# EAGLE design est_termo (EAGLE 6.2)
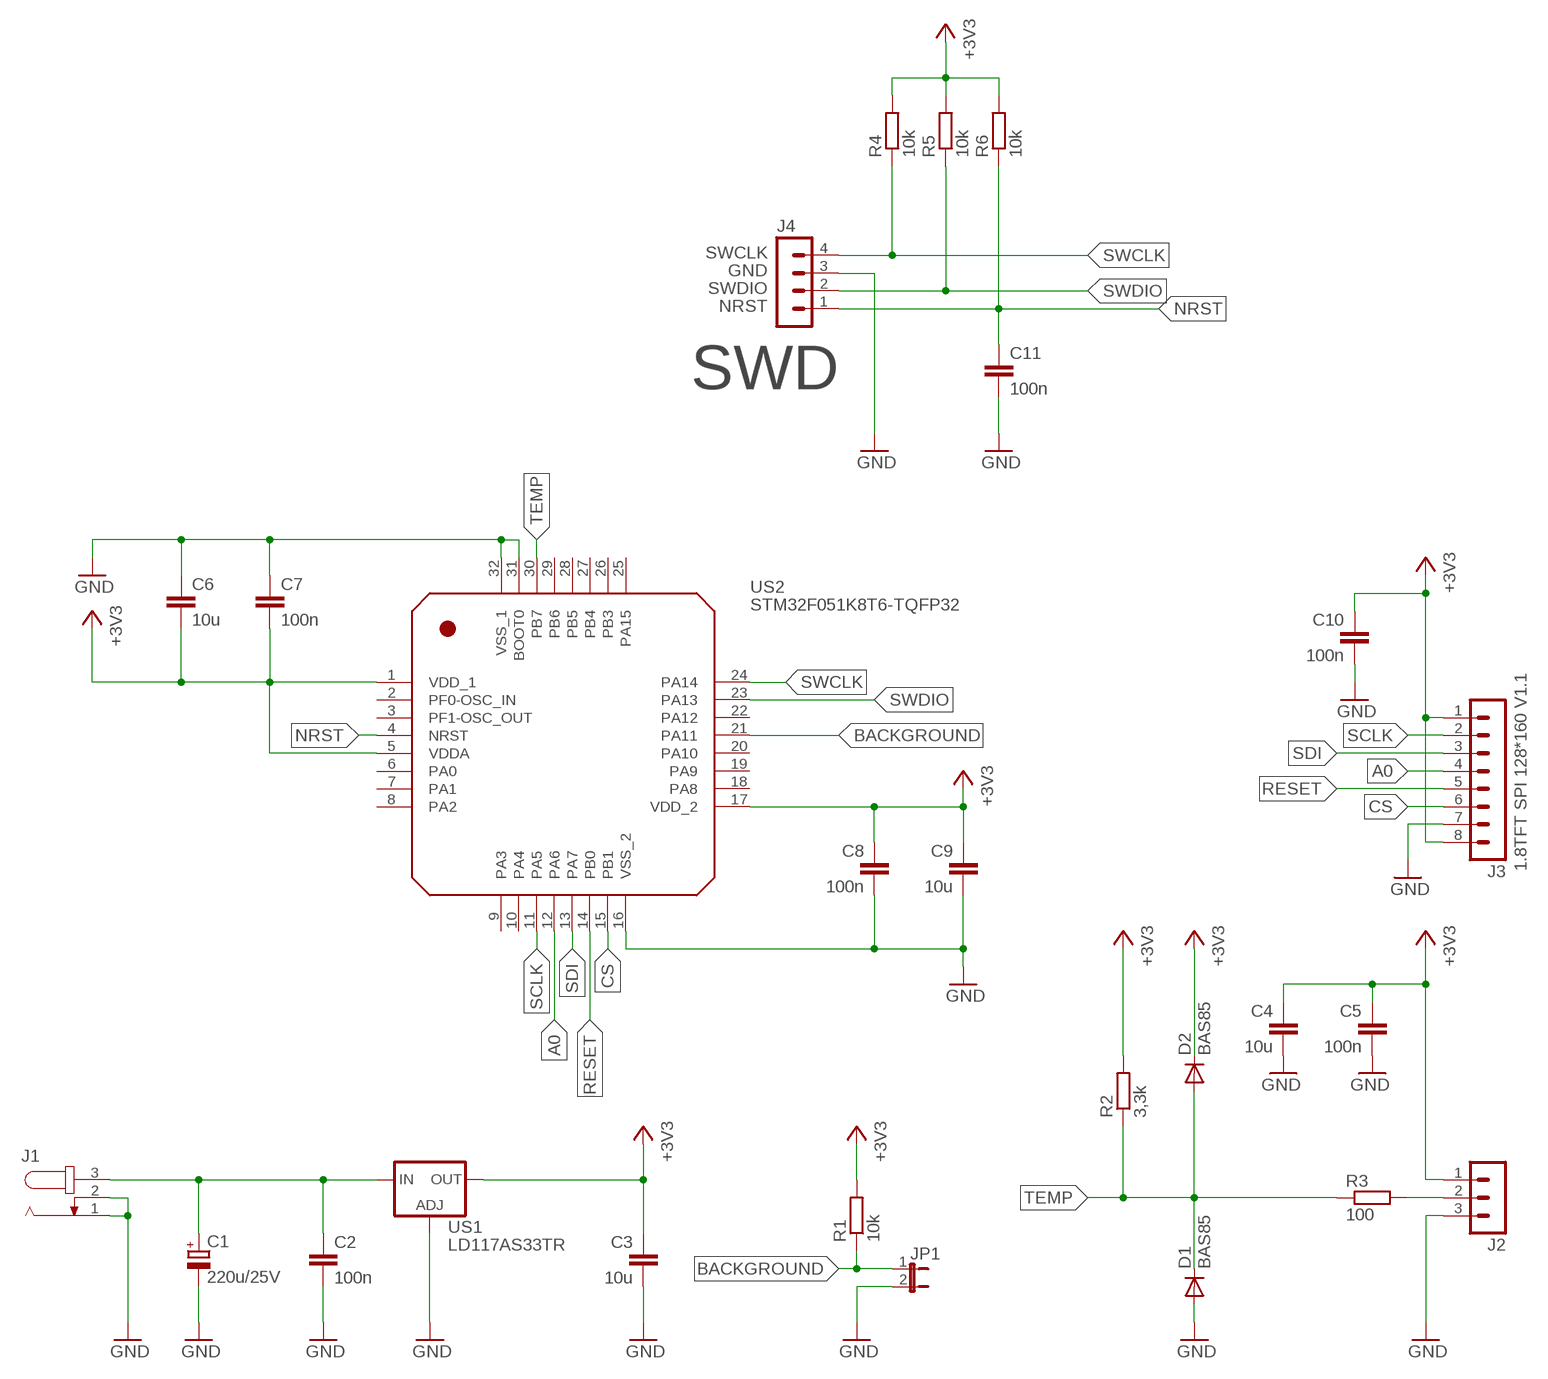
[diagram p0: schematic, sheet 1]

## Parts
C1  220u/25V  CPOL-EUTT2D7L  [TT2D7L]
C2  100n  C-EUC0805  [C0805]
C3  10u  C-EUC0805  [C0805]
C4  10u  C-EUC0805  [C0805]
C5  100n  C-EUC0805  [C0805]
C6  10u  C-EUC0805  [C0805]
C7  100n  C-EUC0805  [C0805]
C8  100n  C-EUC0805  [C0805]
C9  10u  C-EUC0805  [C0805]
C10  100n  C-EUC0805  [C0805]
C11  100n  C-EUC0805  [C0805]
D1  BAS85  DIODE-MINIMELF  [MINIMELF]
D2  BAS85  DIODE-MINIMELF  [MINIMELF]
J1  JACK-PLUG0  [SPC4077]
J2  MA03-1  [MA03-1]
J3  1.8TFT SPI 128*160 V1.1  MA08-1  [MA08-1]
J4  MA04-1  [MA04-1]
JP1  JP1E  [JP1]
R1  10k  R-EU_R0805  [R0805]
R2  3,3k  R-EU_R0805  [R0805]
R3  100  R-EU_R0805  [R0805]
R4  10k  R-EU_R0805  [R0805]
R5  10k  R-EU_R0805  [R0805]
R6  10k  R-EU_R0805  [R0805]
US1  LD117AS33TR  [SOT223]
US2  STM32F051K8T6-TQFP32  STM32F051-TQFP32  [TQFP32]

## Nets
+3V3: C3.1 C4.1 C5.1 C6.2 C7.2 C8.1 C9.1 C10.1 D2.C J2.1 J3.1 J3.8 R1.2 R2.2 R4.2 R5.2 R6.2 US1.4(OUT) US2.1(VDD_1) US2.5(VDDA) US2.17(VDD_2)
A0: J3.4 US2.12(PA6)
BACKGROUND: JP1.1 R1.1 US2.21(PA11)
CS: J3.6 US2.15(PB1)
GND: C1.- C2.2 C3.2 C4.2 C5.2 C6.1 C7.1 C8.2 C9.2 C10.2 C11.2 D1.A J1.1 J1.2 J2.3 J3.7 J4.3 JP1.2 US1.1(ADJ) US2.16(VSS_2) US2.31(BOOT0) US2.32(VSS_1)
N$1: C1.+ C2.1 J1.3 US1.3(IN)
N$28: J2.2 R3.2
NRST: C11.1 J4.1 R6.1 US2.4(NRST)
RESET: J3.5 US2.14(PB0)
SCLK: J3.2 US2.11(PA5)
SDI: J3.3 US2.13(PA7)
SWCLK: J4.4 R4.1 US2.24(PA14)
SWDIO: J4.2 R5.1 US2.23(PA13)
TEMP: D1.C D2.A R2.1 R3.1 US2.30(PB7)
Unconnected: US2.2(PF0-OSC_IN) US2.3(PF1-OSC_OUT) US2.6(PA0) US2.7(PA1) US2.8(PA2) US2.9(PA3) US2.10(PA4) US2.18(PA8) US2.19(PA9) US2.20(PA10) US2.22(PA12) US2.25(PA15) US2.26(PB3) US2.27(PB4) US2.28(PB5) US2.29(PB6)

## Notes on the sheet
- SWCLK
- GND
- SWDIO
- NRST
- SWD

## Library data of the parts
C1 = rcl:CPOL-EU: POLARIZED CAPACITOR, European symbol
C2-C11 = rcl:C-EU: CAPACITOR, European symbol
D1 D2 = diode:DIODE-: DIODE
J1 = con-jack:JACK-PLUG: DC POWER JACK Power Jack, DC, Right Angle, Through Hole, Rated 5A at 16VDC, PC Terminals Distributor: Farnell (www.Farnell.de) Drawing: 84N1161.pdf / 84N1162.pdf Manufacturer: SPC Technology (www.spctechnology.com) Type: SPC4077 / SPC 4078; OC_FARNELL: unknown; OC_NEWARK: unknown
J2 = con-lstb:MA03-1: PIN HEADER; OC_FARNELL: unknown; OC_NEWARK: unknown
J3 = zlacza_futrzak:MA08-1: PIN HEADER; OC_FARNELL: unknown; OC_NEWARK: unknown
J4 = con-lstb:MA04-1: PIN HEADER; OC_FARNELL: unknown; OC_NEWARK: unknown
JP1 = jumper:JP1E: JUMPER
R1-R6 = rcl:R-EU_: RESISTOR, European symbol
US1 = v-reg:LD117A?*: Low drop fixed and adjustable positive voltage regulators 1 A Source: http://www.st.com/stonline/products/literature/ds/7194/ld1117axx.pdf
US2 = scalaki_futrzak:STM32F051-TQFP32

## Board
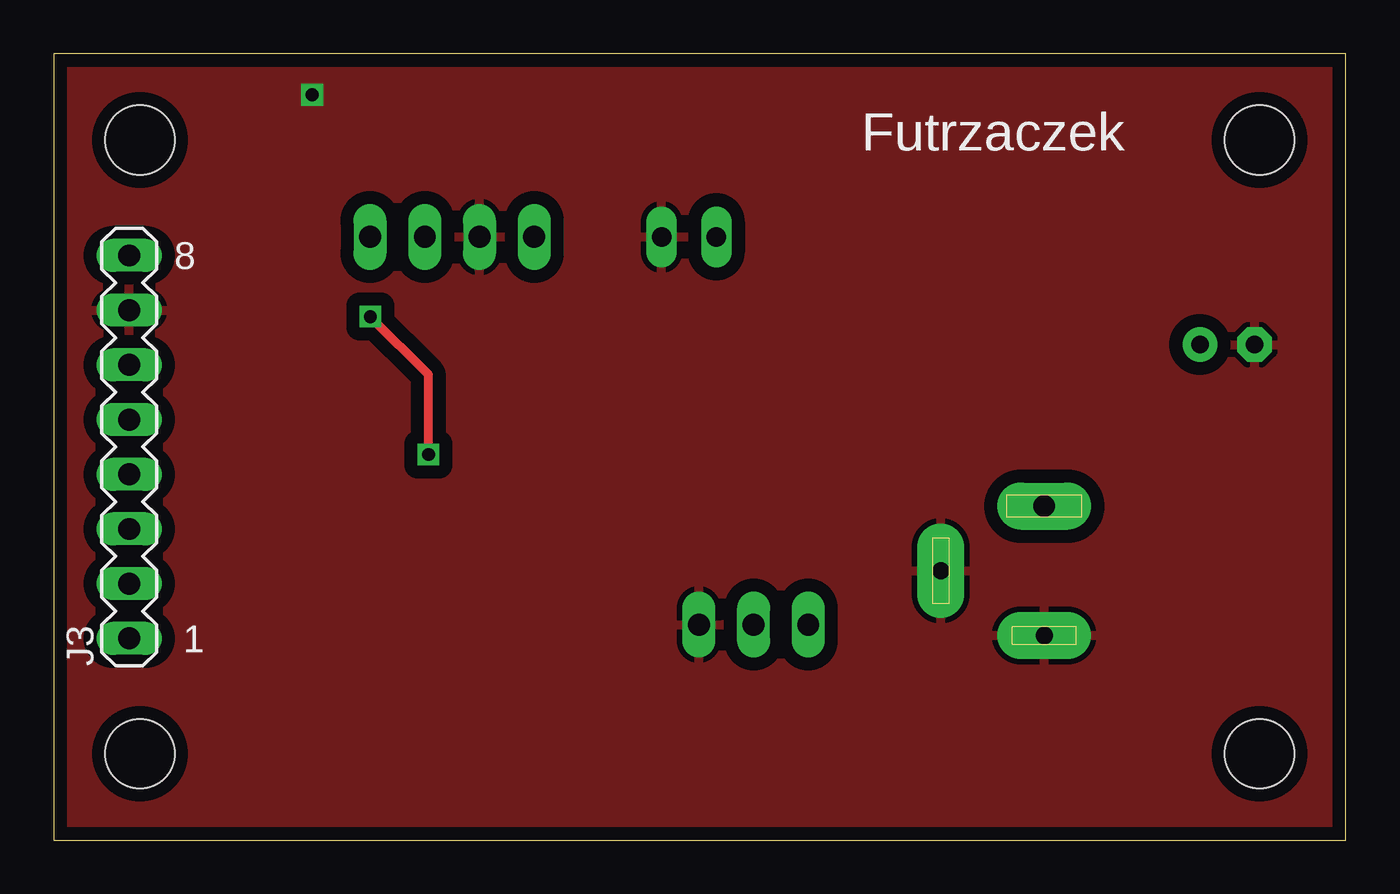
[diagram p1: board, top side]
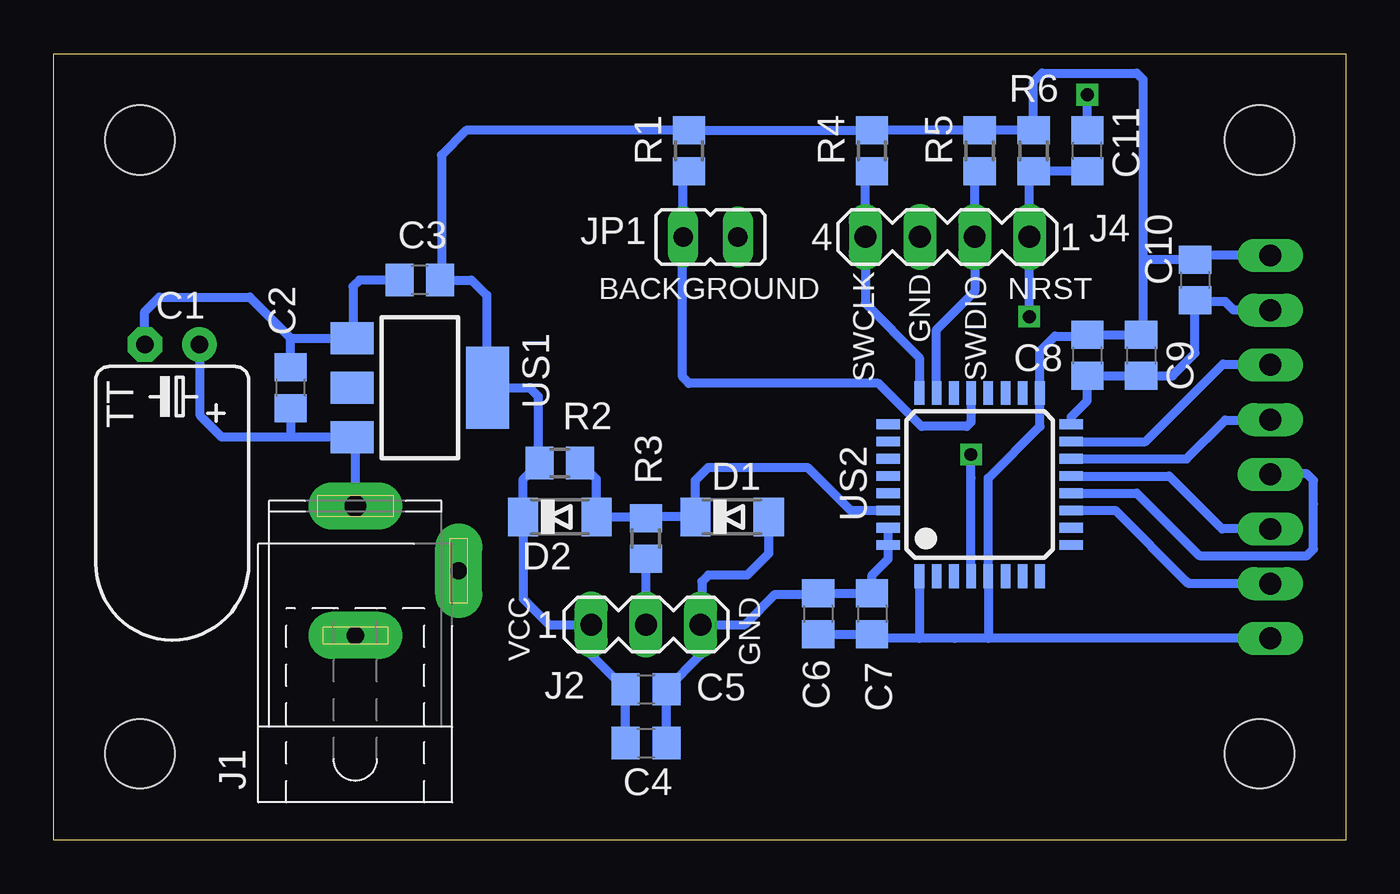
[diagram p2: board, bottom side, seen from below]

Size 60 x 36.5 mm. Coordinates in mm from the lower left corner, seen from the top.
Outline: 0,0 60,0 60,36.5 0,36.5 0,0
Copper layers (1*16): Top 0.035mm / dielectric 1.5mm / Bottom 0.035mm
Design rules: minimum track width 10mil, minimum drill 24mil, track to track 8mil, track to pad 8mil, pad to pad 8mil, via to via 8mil, smd to smd 8mil, copper to edge 20mil, drill to drill 8mil, minimum pad ring 10mil, minimum via ring 8mil, stop-mask expansion 4mil, vias tented up to drill 0mil, thermal gap 10mil
Holes 3.2 mm at 4,4 56,4 4,32.5 56,32.5

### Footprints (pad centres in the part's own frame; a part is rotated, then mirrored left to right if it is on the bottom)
TT2D7L = drill 0.813 pad 1.6: + -1.27,0 | drill 0.813 pad 1.6 octagon: - 1.27,0
C0805 = smd 1.3 x 1.5: 1 -0.95,0; 2 0.95,0
MINIMELF = smd 1.4 x 1.8: A 1.7,0; C -1.7,0
SPC4077 = drill 0.8 pad 2.184 long: 1 -3,0; 2 0,-4.8 | drill 1 pad 2.184 long: 3 3,0
MA03-1 = drill 1.016 long: 1 -2.54,0; 2 0,0; 3 2.54,0
MA08-1 = drill 1.016 long: 1 -8.89,0; 2 -6.35,0; 3 -3.81,0; 4 -1.27,0; 5 1.27,0; 6 3.81,0; 7 6.35,0; 8 8.89,0
MA04-1 = drill 1.016 long: 1 -3.81,0; 2 -1.27,0; 3 1.27,0; 4 3.81,0
JP1 = drill 0.914 long: 1 0,-1.27; 2 0,1.27
R0805 = smd 1.3 x 1.5: 1 -0.95,0; 2 0.95,0
SOT223 = smd 1.5 x 2: 1 -2.3,-3.15; 2 0,-3.15; 3 2.3,-3.15 | smd 3.8 x 2: 4 0,3.15
TQFP32 = smd 1.1 x 0.45: 1 -4.25,2.8; 2 -4.25,2; 3 -4.25,1.2; 4 -4.25,0.4; 5 -4.25,-0.4; 6 -4.25,-1.2; 7 -4.25,-2; 8 -4.25,-2.8; 17 4.25,-2.8; 18 4.25,-2; 19 4.25,-1.2; 20 4.25,-0.4; 21 4.25,0.4; 22 4.25,1.2; 23 4.25,2; 24 4.25,2.8 | smd 0.45 x 1.1: 9 -2.8,-4.25; 10 -2,-4.25; 11 -1.2,-4.25; 12 -0.4,-4.25; 13 0.4,-4.25; 14 1.2,-4.25; 15 2,-4.25; 16 2.8,-4.25; 25 2.8,4.25; 26 2,4.25; 27 1.2,4.25; 28 0.4,4.25; 29 -0.4,4.25; 30 -1.2,4.25; 31 -2,4.25; 32 -2.8,4.25

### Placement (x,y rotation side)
C1  54.5,23 180 bottom
C2  49,21 90 bottom
C3  43,26 180 bottom
C4  32.5,4.5 0 bottom
C5  32.5,7 0 bottom
C6  24.5,10.5 270 bottom
C7  22,10.5 270 bottom
C8  12,22.5 270 bottom
C9  9.5,22.5 270 bottom
C10  7,26 270 bottom
C11  12,32 90 bottom
D1  28.5,15 0 bottom
D2  36.5,15 0 bottom
J1  46,12.5 90 bottom
J2  32.5,10 0 bottom
J3  3.5,18.25 90 top
J4  18.5,28 180 bottom
JP1  29.5,28 270 bottom
R1  30.5,32 90 bottom
R2  36.5,17.5 180 bottom
R3  32.5,14 270 bottom
R4  22,32 90 bottom
R5  17,32 90 bottom
R6  14.5,32 90 bottom
US1  43,21 270 bottom
US2  17,16.5 90 bottom

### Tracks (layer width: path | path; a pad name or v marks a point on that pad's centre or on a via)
+3V3
  Bottom 0.406: C4.1 C5.1 35.04,8.59 J2.1 37,10 38.2,11.2 D2.C 38.2,16.75 R2.2 37.5,17.55 37.5,20.6 37.9,21 US1.4 39.9,21.05 39.9,25.3 40.6,26 C3.1 42,26.05 42,31.8 40.85,32.95 R1.2 R4.2 R5.2 R6.2 14.5,35.2 14.2,35.5 14.1,35.6 9.7,35.6 9.4,35.3 9.4,27 | C6.2 C7.2 21.81,9.36 19.8,9.36 | J3.1 16.6,9.36 | 16.6,9.36 18.16,9.36 19.8,9.36 | US2.1 19.8,9.36 | 16.6,9.36 US2.5 16.6,16.8 14.2,19.2 US2.17 14.2,22.7 13.5,23.4 12.05,23.4 C8.1 C9.1 9.4,23.55 9.4,27 | J3.8 6.81,27.14 C10.1 9.35,26.95 9.4,27
A0
  Bottom 0.406: US2.12 9.7,16.1 7,13.4 6.8,13.2 1.8,13.2 1.5,13.5 1.5,15.6 1.5,16.7 1.8,17 3.48,17 J3.4
BACKGROUND
  Bottom 0.406: R1.1 30.77,30.78 JP1.1 30.8,27.97 30.8,21.5 30.5,21.2 21.7,21.2 19.7,19.2 17.6,19.2 17.4,19.4 US2.21
CS
  Bottom 0.406: US2.15 9.3,18.5 5.7,22.1 3.54,22.1 J3.6
GND  (via drill 0.6)
  Bottom 0.406: C1.- 55.77,24.53 55.1,25.2 50.9,25.2 49.2,23.5 49,23.3 | 49,23.3 US1.1 46.1,23.35 46.1,25.7 45.8,26 C3.2 | C2.2 49,23.3 | J2.3 29.96,8.59 C5.2 C4.2 | J2.3 27.9,10 26.5,11.4 24.55,11.4 C6.1 C7.1 22,12.3 21.3,13 21.25,13.05 US2.32 US2.31 | D1.A 26.8,13.3 27.8,12.3 29.6,12.3 29.9,12 29.9,10.06 J2.3 | US2.16 12.75,19.65 12,20.4 C8.2 C9.2 8.05,21.55 7,22.6 C10.2 6.95,25 5.6,25 5.2,24.6 J3.7 | C11.2 v12,34.6
  pour Top (isolate 0.61): 0,36.5 0,0 60,0 60,36.5
N$1
  Bottom 0.406: J1.3 46,18.5 46.15,18.75 US1.3 49,18.7 | 49,18.7 52.2,18.7 53.2,19.7 53.2,22.97 C1.+ | C2.1 49,18.7
N$28
  Bottom 0.406: J2.2 R3.2
NRST  (via drill 0.6)
  Top 0.406: v17.4,17.9 17.4,21.6 v14.7,24.3
  Bottom 0.406: C11.1 R6.1 14.69,30.86 J4.1 v14.7,24.3 | US2.4 17.4,16.8 v17.4,17.9
RESET
  Bottom 0.406: US2.14 7.4,17.7 5.6,19.5 3.52,19.5 J3.5
SCLK
  Bottom 0.406: US2.11 10.7,15.3 7.4,12 7.3,11.9 J3.2
SDI
  Bottom 0.406: US2.13 8.2,16.9 5.9,14.6 5.74,14.44 J3.3
SWCLK
  Bottom 0.406: R4.1 22.31,30.74 J4.4 22.31,24.91 19.8,22.4 US2.24
SWDIO
  Bottom 0.406: R5.1 17.23,30.82 J4.2 17.23,25.47 17.4,25.3 19,23.7 US2.23
TEMP
  Bottom 0.406: R2.1 34.8,16.75 D2.A 32.55,15 R3.1 32.45,15 D1.C 30.2,16.7 29.6,17.3 25,17.3 23,15.3 US2.30

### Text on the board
tPlace: Futrzaczek | 8 | 1
bPlace: SWDIO | GND | SWCLK | NRST | BACKGROUND | GND | VCC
